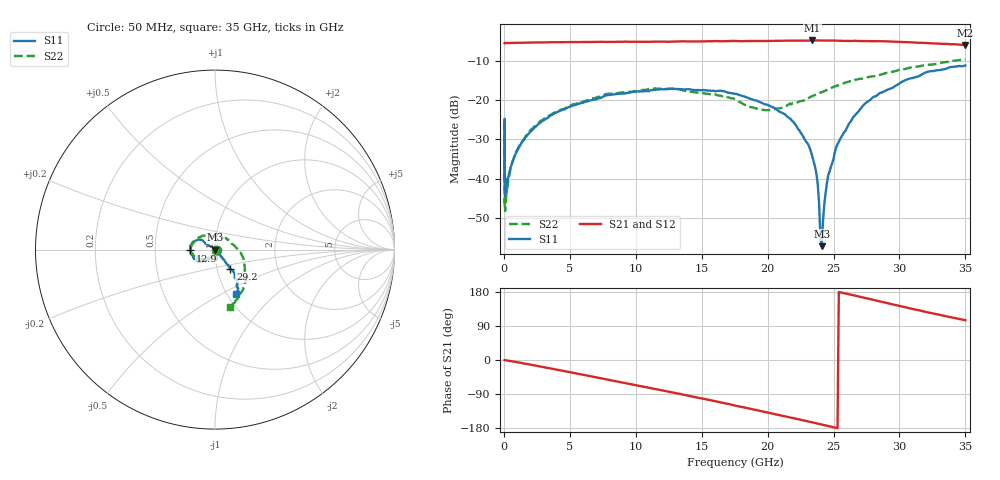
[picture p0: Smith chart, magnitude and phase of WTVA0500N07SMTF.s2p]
! 50 ohm 2-Port S-parameters measured by Modelithics Inc support@modelithics.com  Tampa, FL USA 813-866-6335 (February 2024)
! Smiths Interconnect,  5dB P/N: WTVA0500N07SMTF, Temperature: 25C
! Board: 10 mil Rogers 4350B, Mounting Pad Dimensions: Length: 15 mils, Width: 25 mils, Gap: 40 mils.
# Hz S MA R 50
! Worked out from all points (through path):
!   486 points, 50 MHz to 35 GHz, reference 50 ohm
!   highest |S21| = -4.87 dB at 23.4 GHz (marker M1); lowest = -6.0 dB at 35 GHz (marker M2)
!   group delay of S21, straight-line fit = 20.3 ps
!   lowest |S11| = -57.2 dB at 24.1 GHz (marker M3), VSWR 1.00, Z = 50.1 + j0.00476 ohm
!   |S11| at or under -10 dB: start of sweep to end of sweep
!   |S22| runs from -48.3 to -9.6 dB; largest |S21 - S12| = 0.013
!   S11 on the Smith chart (normalised r, x): 50 MHz: 1.02, -0.01; 12.9 GHz: 0.76, -0.01; 29.2 GHz: 1.16, -0.25; 35 GHz: 1.10, -0.59
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5e7  0.01003 -21.6  0.5281 -0.3  0.528 -0.3  0.004372 -22.2
8e7  0.009598 -31.2  0.5288 -0.4  0.528 -0.4  0.005646 -21.3
9e7  0.005987 -30.5  0.5284 -0.5  0.5282 -0.5  0.003859 -50.9
1.1e8  0.007744 -29.4  0.5285 -0.6  0.5284 -0.6  0.005054 -48.6
7.5e8  0.01817 -88.5  0.5311 -4.3  0.5309 -4.3  0.01825 -99.7
2e9  0.03921 -110.4  0.5361 -12.2  0.5359 -12.2  0.04081 -117.0
5.9e9  0.092 -134.7  0.5446 -38.2  0.5446 -38.2  0.09329 -145.2
1.17e10  0.1354 -171.1  0.5502 -78.1  0.5501 -78.0  0.1393 179.9
1.29e10  0.1377 -178.0  0.5514 -86.3  0.5512 -86.3  0.1391 171.9
1.76e10  0.1195 155.7  0.5617 -121.0  0.5616 -120.8  0.09994 129.3
1.97e10  0.08946 143.9  0.5614 -136.2  0.5612 -136.0  0.07466 94.2
2.15e10  0.06112 147.4  0.5669 -149.7  0.5665 -149.5  0.08574 49.7
2.34e10  0.01884 137.4  0.5705 -164.6  0.5706 -164.4  0.1119 10.2
2.37e10  0.01151 127.3  0.5695 -167.1  0.5694 -166.9  0.1173 5.7
2.39e10  0.004947 120.9  0.5692 -168.7  0.569 -168.4  0.1222 3.3
2.41e10  0.001379 2.0  0.5692 -170.2  0.5689 -170.0  0.1252 0.9
2.42e10  0.002895 -46.0  0.5689 -171.0  0.5688 -170.8  0.1271 -0.5
2.46e10  0.01114 -58.1  0.5693 -174.1  0.5694 -173.9  0.1363 -3.9
2.55e10  0.03193 -49.5  0.5646 178.5  0.5647 178.5  0.1568 -13.6
2.73e10  0.08692 -50.2  0.5614 164.5  0.5613 164.7  0.189 -29.1
2.92e10  0.1371 -51.0  0.5541 149.1  0.5543 149.6  0.222 -40.2
3.5e10  0.2743 -64.9  0.5003 104.9  0.4999 105.2  0.3295 -75.6
